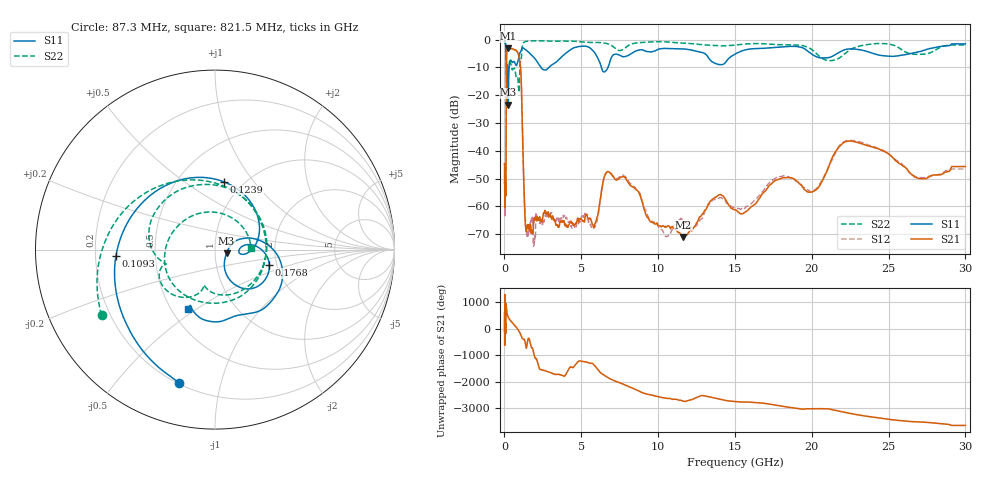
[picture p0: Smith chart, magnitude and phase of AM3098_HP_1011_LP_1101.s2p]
! Date/Time: Thu, Feb 28, 2019 8:43 AM
! Network Analyzer: Agilent Technologies E8364B Rev: A.07.50.67
! Sweep from 0.010 to 30.000 GHz, 1601 Points, Sweep Type: LOG
! Power Supply: 5.023 V, 0.002 A
# Hz S DB R 50
!freq MagS11 AngS11 MagS21 AngS21 MagS12 AngS12 MagS22 AngS22
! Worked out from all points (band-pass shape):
!   1601 points, 10 MHz to 30 GHz, reference 50 ohm
!   highest |S21| = -3.14 dB at 262.5 MHz (marker M1); lowest = -71.1 dB at 11.65 GHz (marker M2)
!   |S21| within 3 dB of the highest: 137.5 MHz to 945 MHz (807.5 MHz wide, 149 % of centre)
!   lowest |S11| = -23.4 dB at 242.3 MHz (marker M3), VSWR 1.14, Z = 56.8 - j2.39 ohm
!   |S11| at or under -10 dB: 192.4 MHz to 303 MHz (110.6 MHz wide, 44.6 % of centre); 2.372 GHz to 2.902 GHz (530.5 MHz wide, 20.1 % of centre); 6.303 GHz to 6.74 GHz (436.6 MHz wide, 6.7 % of centre)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
!   |S22| runs from -19.0 to -0.4 dB; largest |S21 - S12| = 0.011
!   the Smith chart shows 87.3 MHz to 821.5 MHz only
!   S11 on the Smith chart (normalised r, x): 87.3 MHz: 0.21, -0.74; 109.3 MHz: 0.29, -0.03; 123.9 MHz: 0.81, +0.72; 176.8 MHz: 1.83, -0.34; 821.5 MHz: 0.61, -0.46
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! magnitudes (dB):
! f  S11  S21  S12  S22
! 10 MHz  -0.3  -44.8  -44.7  -0.6
! 38.04 MHz  -0.4  -59.8  -59.8  -0.9
! 87.3 MHz  -2.3  -54.3  -54.7  -2.7
! 98.44 MHz  -3.6  -51.7  -51.7  -4.0
! 109.3 MHz  -5.1  -33.9  -33.7  -6.4
! 123.9 MHz  -8.4  -13.6  -13.5  -10.8
! 144.7 MHz  -17.4  -5.1  -5.0  -13.7
! 176.8 MHz  -10.1  -3.9  -3.9  -9.4
! 242.3 MHz  -23.4  -3.2  -3.1  -10.9
! 262.5 MHz  -16.9  -3.1  -3.1  -10.5
! 550.5 MHz  -8.1  -3.5  -3.4  -10.7
! 821.5 MHz  -8.8  -4.3  -4.3  -13.9
! 1.071 GHz  -4.3  -12.0  -12.0  -7.7
! 1.389 GHz  -3.7  -68.1  -67.3  -0.7
! 2.084 GHz  -7.6  -64.0  -62.8  -0.4
! 5.783 GHz  -4.1  -67.1  -67.3  -1.0
! 6.653 GHz  -10.9  -47.7  -47.7  -1.4
! 7.926 GHz  -6.0  -50.3  -49.7  -2.7
! 11.65 GHz  -3.4  -71.1  -64.9  -1.3
! 20 GHz  -5.3  -54.9  -54.8  -3.6
! 22.56 GHz  -3.4  -36.5  -36.3  -3.5
! 30 GHz  -1.6  -45.7  -46.6  -1.9
